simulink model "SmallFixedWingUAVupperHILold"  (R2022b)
settings: Solver=FixedStepDiscrete  StartTime=0.0  StopTime=inf  FixedStep=1/150  RelTol=1e-3
model workspace: external: MAT-File (data not in the file)
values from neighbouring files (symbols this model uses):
  env = struct    [InitDatactrl.m]
  uav = struct    [InitDatactrl.m]    (also in InitDatactrldf.m)
  x = x + points(1, i) * k(i) * ft    [bezir_n.m]
undefined symbols (not defined in the file or in its folder): current_a, current_filtered_a, DiscIntNeverNeededParam, remaining, RGBLED_COLOR_ENUM, RGBLED_MODE_ENUM, voltage_filtered_v, voltage_v
libraries: simulink x10, pixhawk_slib_sensors_actuators x6, pixhawk_slib_uORB_RW x5

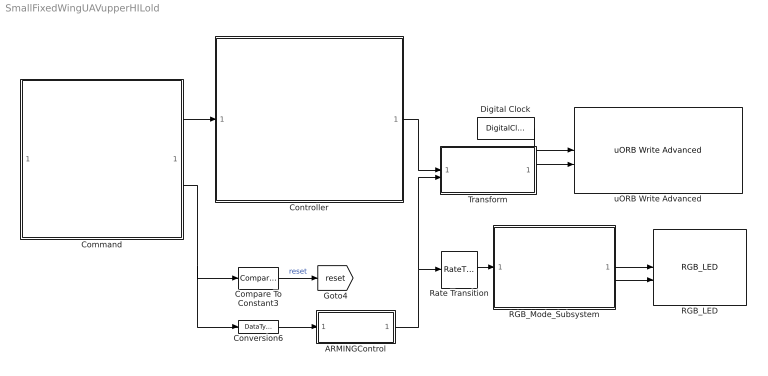
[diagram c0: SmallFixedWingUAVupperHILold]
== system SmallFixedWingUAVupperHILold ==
  ARMINGControl : Subsystem
  Command : Subsystem
  Compare To Constant3 : simulink/Logic and Bit Operations/Compare To Constant  relop=<=  const=1100  OutDataTypeStr=boolean
  Controller : Subsystem
  Conversion6 : DataTypeConversion  OutDataTypeStr=double
  Digital Clock : DigitalClock  SampleTime=-1
  RGB_LED : pixhawk_slib_sensors_actuators/RGB_LED
  RGB_Mode_Subsystem : Subsystem
  Rate Transition : RateTransition  OutPortSampleTime=1
  Transform : Subsystem
  uORB Write Advanced : pixhawk_slib_uORB_RW/uORB Write Advanced  Ts=0  uORB_AdvtQueue=on  uORB_FieldEnabledArr="0  0  0  1  0  0  0  0  0  0  0"  uORB_Topic_str=0  uORB_Struct_DT="[1  1  1  1  1]"  BlockInputCount=5  uORB_StructParams="[\"voltage_v\",\"voltage_filtered_v\",\"current_a\",\"current_filtered_a\",\"remaining\"]"  uORB_PortSizes="[1  1  1  1]"  MsgSizeOf=0  MW_update=true
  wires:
  Digital Clock/1 -> uORB Write Advanced/1
  RGB_Mode_Subsystem/1(RGB_MODE) -> RGB_LED/1
  Rate Transition/1 -> RGB_Mode_Subsystem/1(ARM_STATE)
  ARMINGControl/1(Out1) -> Transform/2(Arm), Rate Transition/1
  RGB_Mode_Subsystem/2(RGB_COLOR) -> RGB_LED/2
  Conversion6/1 -> ARMINGControl/1(In1)
  Compare To Constant3/1 -> [reset]  "reset"
  Transform/1(PWMOuput) -> uORB Write Advanced/2
  Controller/1(Actuator) -> Transform/1(ActuatorCmd)
  Command/2(Arm) -> Conversion6/1, Compare To Constant3/1
  Command/1(Command) -> Controller/1(Command)

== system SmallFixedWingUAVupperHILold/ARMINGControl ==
  In1 : Inport
  Compare To Constant3 : simulink/Logic and Bit Operations/Compare To Constant  relop=>=  const=uint16(1500)  OutDataTypeStr=boolean
  Out1 : Outport  VectorParamsAs1DForOutWhenUnconnected=off
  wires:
  Compare To Constant3/1 -> Out1/1
  In1/1 -> Compare To Constant3/1

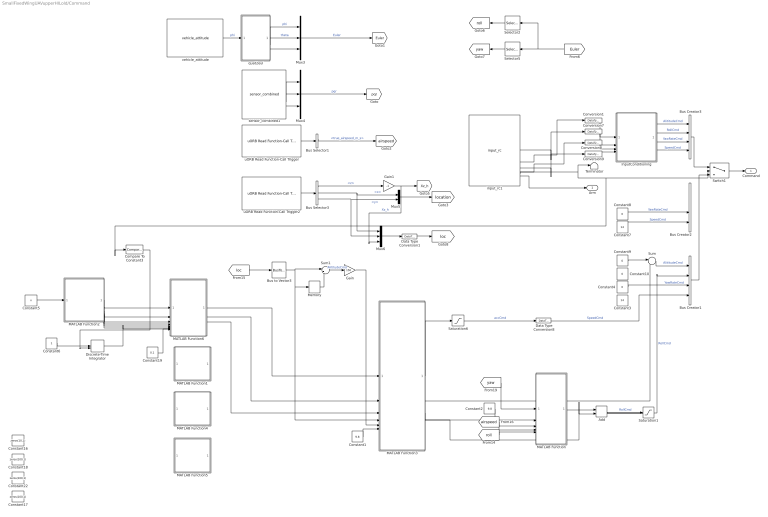
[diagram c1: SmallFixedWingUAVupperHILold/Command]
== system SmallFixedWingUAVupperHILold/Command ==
  Add : Sum
  Bus Creator1 : BusCreator  Inputs=4
  Bus Creator2 : BusCreator  Inputs=4
  Bus Creator3 : BusCreator  Inputs=4
  Bus Selector1 : BusSelector  OutputSignals=true_airspeed_m_s
  Bus Selector3 : BusSelector  OutputSignals=z,x,y
  Bus to Vector3 : BusToVector
  Compare To Constant3 : simulink/Logic and Bit Operations/Compare To Constant  relop=>=  const=uint16(1500)  OutDataTypeStr=boolean
  Constant1 : Constant  Value=9.8
  Constant{4,8..10} (4 alike) : Constant  Value=0  SampleTime=-1
  Constant16 : Constant  Value=zeros(10,1)
  Constant17 : Constant  Value=zeros(100,1)
  Constant18 : Constant  Value=zeros(100,1)
  Constant19 : Constant  Value=0.1
  Constant2 : Constant  Value=9.8  SampleTime=-1
  Constant22 : Constant  Value=zeros(100,1)
  Constant3 : Constant  Value=14  SampleTime=-1
  Constant5 : Constant  Value=x
  Constant6 : Constant
  Constant7 : Constant  Value=14  SampleTime=-1
  Conversion{1,7..9} (4 alike) : DataTypeConversion  OutDataTypeStr=double
  Data Type Conversion1 : DataTypeConversion  OutDataTypeStr=double
  Data Type Conversion8 : DataTypeConversion  OutDataTypeStr=single
  Discrete-Time Integrator : DiscreteIntegrator  ExternalReset=either  SampleTime=-1  ICPrevOutput=DiscIntNeverNeededParam  ICPrevScaledInput=DiscIntNeverNeededParam
  Gain : Gain  Gain=150
  Gain1 : Gain  Gain=-1
  InputConditioning : Subsystem
  MATLAB Function : MATLAB Function  TreatAsAtomicUnit=on
  MATLAB Function1 : MATLAB Function  Commented=on  TreatAsAtomicUnit=on
  MATLAB Function2 : MATLAB Function  TreatAsAtomicUnit=on
  MATLAB Function3 : MATLAB Function  TreatAsAtomicUnit=on
  MATLAB Function4 : MATLAB Function  Commented=on  TreatAsAtomicUnit=on
  MATLAB Function5 : MATLAB Function  Commented=on  TreatAsAtomicUnit=on
  MATLAB Function6 : MATLAB Function  TreatAsAtomicUnit=on
  Memory : Memory  InheritSampleTime=on
  Mux3 : Mux  Inputs=3
  Mux4 : Mux  Inputs=3
  Mux5 : Mux  Inputs=2
  Mux6 : Mux  Inputs=3
  Saturation1 : Saturate  UpperLimit=0.4  LowerLimit=-0.4
  Saturation6 : Saturate  UpperLimit=10  LowerLimit=-10
  Selector2 : Selector  InputPortWidth=3  IndexOptions=Index vector (dialog)  Indices=1  OutputSizes=1
  Selector5 : Selector  InputPortWidth=3  IndexOptions=Index vector (dialog)  Indices=3  OutputSizes=1
  Sum : Sum  Inputs=|++
  Sum1 : Sum  Inputs=|+-
  Switch1 : Switch  Criteria=u2 > Threshold  Threshold=1500
  Terminator : Terminator
  input_rc1 : pixhawk_slib_sensors_actuators/input_rc  Description=|  sampletime=1/150  channel1=on  channel2=on  channel3=on  channel4=on  channel5=on  channel6=on  channel7=off  channel8=off  channel9=off  channel10=off  channel11=off  channel12=off  channel13=off  channel14=off  channel15=off  channel16=off  channel17=off  channel18=off  ch_count=off  rssi=off  rc_failsafe=off  rc_lost=off  rc_inputsource=off
      | RC Input Block
      | 
      | This block provides user input control to the model.
      | It uses the input_rc uORB topic.
      | 
      | The user has the ability to choose which channels are available as outputs from this block and also some optional outputs. These include 
      | Channels 1 through 18
      | double data type indicating the PWM value from the controller 
      | measured pulse widths for each of the supported channels 
      | Channel Count 
      | u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
  quat2eul : MATLAB Function  TreatAsAtomicUnit=on
  sensor_combined1 : pixhawk_slib_sensors_actuators/sensor_combined  Description=|  sampletime=1/150  show_mag=off  show_acc=off  show_gyro=on  show_baro=off  show_ts=off
      | Sensor Combined Block
      | 
      | This block enables access to the various sensors available on the px4fmu-v2 hardware.  
      | The user can use these signals in the Simulink control model.  
      | The sample time needs to be provided in the mask dialog.  
      | Optional output ports can also be selected.  
      | Refer to the sample model: px4demo_attitude_control.slx
      | 
      | Signal definitions: 
      | Magnetometer (x,y,z) - single values – Mag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
  uORB Read Function-Call Trigger : pixhawk_slib_uORB_RW/uORB Read Function-Call Trigger  uORB_Topic_str='airspeed'  BusObjVar=Bus: airspeed_SL  uORB_Interval=1  AsyncOutput=off  Fcn_call_select=Generate Function Call Signal  TaskName='Task1'  Poll_timeout=100  Ts=-1
  uORB Read Function-Call Trigger2 : pixhawk_slib_uORB_RW/uORB Read Function-Call Trigger  uORB_Topic_str='vehicle_local_position'  BusObjVar=Bus: vehicle_local_position_SL  uORB_Interval=1  AsyncOutput=off  Fcn_call_select=Generate Function Call Signal  TaskName='Task1'  Poll_timeout=100  Ts=-1
  vehicle_attitude : pixhawk_slib_sensors_actuators/vehicle_attitude  sampletime=1/150  show_r=off  show_p=off  show_y=off  show_q=on  show_ts=off
  Command : Outport  VectorParamsAs1DForOutWhenUnconnected=off
  Arm : Outport  Port=2  VectorParamsAs1DForOutWhenUnconnected=off
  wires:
  InputConditioning/3(yawRate_d) -> Bus Creator3/3  "YawRateCmd"
  Conversion9/1 -> InputConditioning/4(ch4)
  InputConditioning/2(Roll_d) -> Bus Creator3/2  "RollCmd"
  Constant8/1 -> Bus Creator2/3  "YawRateCmd"
  InputConditioning/4(Speed_d) -> Bus Creator3/4  "SpeedCmd"
  Conversion1/1 -> InputConditioning/1("ch1 ")
  InputConditioning/1(Altitude_d) -> Bus Creator3/1  "AlititudeCmd"
  input_rc1/5 -> Switch1/2, Compare To Constant3/1, Terminator/1
  Conversion8/1 -> InputConditioning/3(ch3)
  Constant7/1 -> Bus Creator2/4  "SpeedCmd"
  Bus Creator3/1 -> Switch1/1
  Conversion7/1 -> InputConditioning/2(ch2)
  Switch1/1 -> Command/1
  input_rc1/6 -> Arm/1
  MATLAB Function3/4(roll) -> Add/2
  Saturation6/1 -> Data Type Conversion8/1  "accCmd"
  [airspeed] -> MATLAB Function/4(V)
  MATLAB Function3/3(yaw) -> MATLAB Function/2(yawdes)
  Bus to Vector3/1 -> Sum1/1, Memory/1, MATLAB Function3/4(x)
  Constant2/1 -> MATLAB Function/3(g)
  Constant1/1 -> MATLAB Function3/6(g)
  MATLAB Function/1(roll) -> Add/1
  MATLAB Function3/1(av1) -> Saturation6/1
  [loc] -> Bus to Vector3/1
  [roll] -> MATLAB Function/5(rolldes)
  [yaw] -> MATLAB Function/1(yaw)
  sensor_combined1/3 -> Mux4/3
  Mux4/1 -> [pqr]  "pqr"
  Mux3/1 -> [Euler]  "Euler"
  quat2eul/1(phi) -> Mux3/1  "phi"
  uORB Read Function-Call Trigger/1 -> Bus Selector1/1
  Bus Selector1/1 -> [airspeed]  "<true_airspeed_m_s>"
  vehicle_attitude/1 -> quat2eul/1(q)  "phi"
  quat2eul/2(theta) -> Mux3/2  "theta"
  sensor_combined1/2 -> Mux4/2
  sensor_combined1/1 -> Mux4/1
  quat2eul/3(psi) -> Mux3/3
  Mux6/1 -> Data Type Conversion1/1
  Bus Selector3/2 -> Mux6/1, Mux5/1  "<x>"
  Bus Selector3/3 -> Mux6/2, Mux5/2  "<y>"
  Bus Selector3/1 -> Gain1/1  "<z>"
  Gain1/1 -> Mux6/3, [Xz_h]  "Xz_h"
  Mux5/1 -> [location]
  uORB Read Function-Call Trigger2/1 -> Bus Selector3/1
  Data Type Conversion1/1 -> [loc]
  Selector2/1 -> [roll]
  Selector5/1 -> [yaw]
  [Euler] -> Selector2/1, Selector5/1
  Add/1 -> Saturation1/1  "RollCmd"
  Sum/1 -> Bus Creator1/1  "AlititudeCmd"
  Constant4/1 -> Bus Creator1/3  "YawRateCmd"
  Constant9/1 -> Sum/1
  Data Type Conversion8/1 -> Bus Creator1/4  "SpeedCmd"
  Memory/1 -> Sum1/2
  Sum1/1 -> Gain/1  "AlititudeCmd"
  Gain/1 -> MATLAB Function3/5(dx)
  Constant5/1 -> MATLAB Function2/1(x)
  MATLAB Function3/2(Hz) -> Sum/2
  Constant19/1 -> MATLAB Function6/8(sample_tt)
  MATLAB Function2/1(xx) -> MATLAB Function6/1(x)
  MATLAB Function6/1(xdx) -> MATLAB Function3/1(xd)
  MATLAB Function6/2(vdv) -> MATLAB Function3/2(dxd)
  MATLAB Function6/3(ada) -> MATLAB Function3/3(ddxd)
  Constant6/1 -> Discrete-Time Integrator/1
  Discrete-Time Integrator/1 -> MATLAB Function6/7(t)
  MATLAB Function2/2(y) -> MATLAB Function6/2(y)
  MATLAB Function2/3(dx) -> MATLAB Function6/3(dx)
  MATLAB Function2/4(dy) -> MATLAB Function6/4(dy)
  MATLAB Function2/5(ddx) -> MATLAB Function6/5(ddx)
  MATLAB Function2/6(ddy) -> MATLAB Function6/6(ddy)
  Saturation1/1 -> Bus Creator1/2  "RollCmd"
  Compare To Constant3/1 -> Discrete-Time Integrator/2
  Bus Creator1/1 -> Switch1/3
  input_rc1/3 -> Conversion9/1
  input_rc1/4 -> Conversion8/1
  input_rc1/1 -> Conversion7/1
  input_rc1/2 -> Conversion1/1

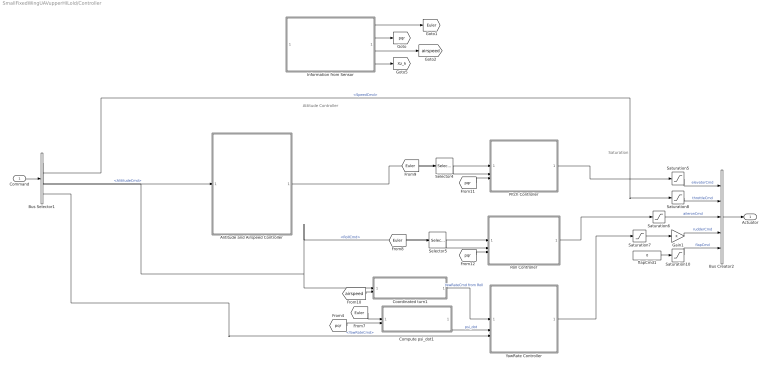
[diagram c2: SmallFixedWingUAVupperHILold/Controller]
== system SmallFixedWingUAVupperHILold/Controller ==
  note: Saturation
  note: Attitude Controller
  Command : Inport
  Alititude and Airspeed Controller : Subsystem
  Bus Creator2 : BusCreator  Inputs=5
  Bus Selector1 : BusSelector  OutputSignals=AlititudeCmd,SpeedCmd,RollCmd,YawRateCmd
  Compute psi_dot1 : Subsystem
  Coordinated turn1 : Subsystem
  Gain1 : Gain
  Information from Sensor : Subsystem
  Pitch Controller : Subsystem
  Roll Controller : Subsystem
  Saturation10 : Saturate  UpperLimit=uav.flap.max  LowerLimit=uav.flap.min
  Saturation5 : Saturate  UpperLimit=uav.elevator.max  LowerLimit=uav.elevator.min
  Saturation6 : Saturate  UpperLimit=uav.aileron.max  LowerLimit=uav.aileron.min
  Saturation7 : Saturate  UpperLimit=uav.rudder.max  LowerLimit=uav.rudder.min
  Saturation8 : Saturate  UpperLimit=uav.throttlepercent.max  LowerLimit=uav.throttlepercent.min
  Selector4 : Selector  InputPortWidth=3  IndexOptions=Index vector (dialog)  Indices=2  OutputSizes=1
  Selector5 : Selector  InputPortWidth=3  IndexOptions=Index vector (dialog)  Indices=1  OutputSizes=1
  YawRate Controller : Subsystem
  flapCmd1 : Constant  Value=0  OutDataTypeStr=double
  Actuator : Outport
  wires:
  Information from Sensor/1(Euler) -> [Euler]
  Information from Sensor/3(<true_airspeed_m_s>) -> [airspeed]
  Information from Sensor/2(pqr) -> [pqr]
  Information from Sensor/4(Xz_h) -> [Xz_h]
  Gain1/1 -> Bus Creator2/4  "rudderCmd"
  [pqr] -> Pitch Controller/3(pqr)
  [airspeed] -> Coordinated turn1/2(<airpseed>)
  Roll Controller/1(aileronCmd) -> Saturation6/1
  Bus Selector1/1 -> Alititude and Airspeed Controller/1(<AlititudeCmd>)  "<AlititudeCmd>"
  Saturation7/1 -> Gain1/1
  Bus Selector1/3 -> Coordinated turn1/1(<RollCmd>), Roll Controller/1(Roll cmd)  "<RollCmd>"
  Coordinated turn1/1(YawRateCmd) -> YawRate Controller/1(psi_dot Cmd)  "YawRateCmd from Roll"
  [Euler] -> Selector4/1
  Alititude and Airspeed Controller/1(pitchout) -> Pitch Controller/1(Pitch cmd)
  Pitch Controller/1(elevatorCmd) -> Saturation5/1
  Saturation8/1 -> Bus Creator2/2  "throttleCmd"
  Command/1 -> Bus Selector1/1
  flapCmd1/1 -> Saturation10/1
  Compute psi_dot1/1(psi_dot) -> YawRate Controller/2(psi_dot)  "psi_dot"
  [Euler] -> Selector5/1
  Bus Selector1/4 -> YawRate Controller/3(<YawRateCmd>)  "<YawRateCmd>"
  Saturation6/1 -> Bus Creator2/3  "aileronCmd"
  [pqr] -> Compute psi_dot1/2(G)
  Selector4/1 -> Pitch Controller/2(Pitch act)
  YawRate Controller/1(rudderCmd) -> Saturation7/1
  [pqr] -> Roll Controller/3(pqr)
  Selector5/1 -> Roll Controller/2(Roll act)
  Saturation5/1 -> Bus Creator2/1  "elevatorCmd"
  [Euler] -> Compute psi_dot1/1(Euler)
  Saturation10/1 -> Bus Creator2/5  "flapCmd"
  Bus Creator2/1 -> Actuator/1
  Bus Selector1/2 -> Saturation8/1  "<SpeedCmd>"

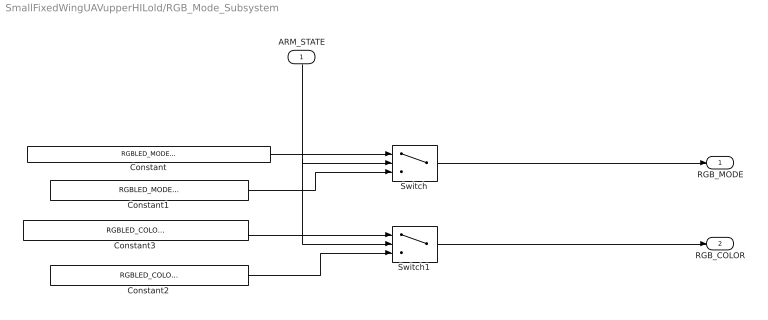
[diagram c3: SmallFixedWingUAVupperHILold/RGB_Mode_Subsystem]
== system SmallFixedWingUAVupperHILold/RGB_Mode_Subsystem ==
  ARM_STATE : Inport
  Constant : Constant  Value=RGBLED_MODE_ENUM.SL_MODE_BLINK_FAST  OutDataTypeStr=Enum: RGBLED_MODE_ENUM
  Constant1 : Constant  Value=RGBLED_MODE_ENUM.SL_MODE_BREATHE  OutDataTypeStr=Enum: RGBLED_MODE_ENUM
  Constant2 : Constant  Value=RGBLED_COLOR_ENUM.SL_COLOR_GREEN  OutDataTypeStr=Enum: RGBLED_COLOR_ENUM
  Constant3 : Constant  Value=RGBLED_COLOR_ENUM.SL_COLOR_BLUE  OutDataTypeStr=Enum: RGBLED_COLOR_ENUM
  Switch : Switch  Criteria=u2 ~= 0  Threshold=1500
  Switch1 : Switch  Criteria=u2 ~= 0  Threshold=1500
  RGB_MODE : Outport  VectorParamsAs1DForOutWhenUnconnected=off
  RGB_COLOR : Outport  Port=2  VectorParamsAs1DForOutWhenUnconnected=off
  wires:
  ARM_STATE/1 -> Switch1/2, Switch/2
  Constant/1 -> Switch/1
  Constant1/1 -> Switch/3
  Switch/1 -> RGB_MODE/1
  Constant3/1 -> Switch1/1
  Constant2/1 -> Switch1/3
  Switch1/1 -> RGB_COLOR/1

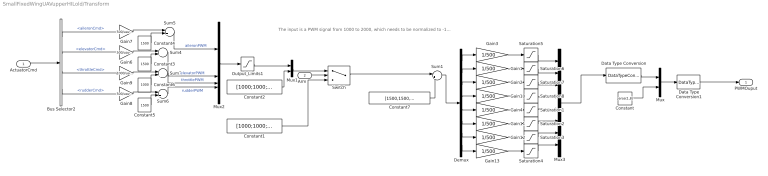
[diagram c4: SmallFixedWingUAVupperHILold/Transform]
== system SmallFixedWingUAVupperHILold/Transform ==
  note: The input is a PWM signal from 1000 to 2000, which needs to be normalized to -1~1.
  ActuatorCmd : Inport
  Arm : Inport  Port=2
  Bus Selector2 : BusSelector  OutputSignals=aileronCmd,elevatorCmd,throttleCmd,rudderCmd
  Constant : Constant  Value=zeros(1,8)
  Constant1 : Constant  Value=[1000;1000;1000;1000;1000;1000;1000;1000]
  Constant2 : Constant  Value=[1000;1000;1000;1000]
  Constant3 : Constant  Value=1500
  Constant4 : Constant  Value=1500
  Constant5 : Constant  Value=1500
  Constant6 : Constant  Value=1000
  Constant7 : Constant  Value=[1500,1500,1500,1500,1500,1500,1500,1500]
  Data Type Conversion : DataTypeConversion  OutDataTypeStr=double
  Data Type Conversion1 : DataTypeConversion  OutDataTypeStr=single
  Demux : Demux  Outputs=8
  Gain{1..4,10..13} (8 alike) : Gain  Gain=1/500
  Gain6 : Gain  Gain=500/uav.controlsurfacemax
  Gain7 : Gain  Gain=500/uav.controlsurfacemax
  Gain8 : Gain  Gain=500/uav.controlsurfacemax
  Gain9 : Gain  Gain=1000/uav.throttlepercent.max
  Mux : Mux  Inputs=2
  Mux1 : Mux  Inputs=2
  Mux2 : Mux
  Mux3 : Mux  Inputs=8
  Output_Limits1 : Saturate  UpperLimit=2000  LowerLimit=1000
  Saturation{1..8} (8 alike) : Saturate  UpperLimit=1  LowerLimit=-1
  Sum1 : Sum  Inputs=|+-
  Sum{4..7} (4 alike) : Sum  Inputs=|++
  Switch : Switch  Criteria=u2 > Threshold  Threshold=0.5
  PWMOuput : Outport  VectorParamsAs1DForOutWhenUnconnected=off
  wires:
  Constant2/1 -> Mux1/2
  Sum6/1 -> Mux2/4  "rudderPWM"
  Data Type Conversion/1 -> Mux/1
  Bus Selector2/4 -> Gain8/1  "<rudderCmd>"
  Bus Selector2/2 -> Gain6/1  "<elevatorCmd>"
  Constant3/1 -> Sum4/2
  Gain6/1 -> Sum4/1
  Bus Selector2/3 -> Gain9/1  "<throttleCmd>"
  Bus Selector2/1 -> Gain7/1  "<aileronCmd>"
  Constant/1 -> Mux/2
  Gain8/1 -> Sum6/1
  Sum7/1 -> Mux2/3  "throttlePWM"
  Constant1/1 -> Switch/3
  Mux1/1 -> Switch/1
  Output_Limits1/1 -> Mux1/1
  Constant5/1 -> Sum6/2
  Sum5/1 -> Mux2/1  "aileronPWM"
  Sum4/1 -> Mux2/2  "elevatorPWM"
  Constant6/1 -> Sum7/2
  Mux2/1 -> Output_Limits1/1
  Gain7/1 -> Sum5/1
  Mux/1 -> Data Type Conversion1/1
  Gain9/1 -> Sum7/1
  Constant4/1 -> Sum5/2
  Arm/1 -> Switch/2
  ActuatorCmd/1 -> Bus Selector2/1
  Data Type Conversion1/1 -> PWMOuput/1
  Demux/1 -> Gain3/1
  Saturation6/1 -> Mux3/2
  Saturation5/1 -> Mux3/1
  Gain1/1 -> Saturation6/1
  Sum1/1 -> Demux/1
  Saturation8/1 -> Mux3/4
  Gain2/1 -> Saturation7/1
  Demux/4 -> Gain10/1
  Gain3/1 -> Saturation5/1
  Demux/2 -> Gain1/1
  Saturation7/1 -> Mux3/3
  Demux/3 -> Gain2/1
  Gain10/1 -> Saturation8/1
  Constant7/1 -> Sum1/2
  Demux/7 -> Gain12/1
  Demux/6 -> Gain11/1
  Demux/5 -> Gain4/1
  Demux/8 -> Gain13/1
  Gain4/1 -> Saturation1/1
  Saturation1/1 -> Mux3/5
  Gain11/1 -> Saturation2/1
  Saturation2/1 -> Mux3/6
  Gain12/1 -> Saturation3/1
  Saturation3/1 -> Mux3/7
  Gain13/1 -> Saturation4/1
  Saturation4/1 -> Mux3/8
  Switch/1 -> Sum1/1
  Mux3/1 -> Data Type Conversion/1

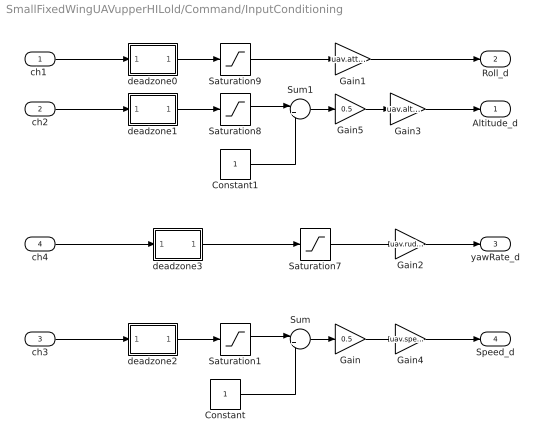
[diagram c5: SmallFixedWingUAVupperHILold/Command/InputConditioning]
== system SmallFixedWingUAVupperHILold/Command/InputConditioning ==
  "ch1 " : Inport
  ch2 : Inport  Port=2
  ch3 : Inport  Port=3
  ch4 : Inport  Port=4
  Constant : Constant
  Constant1 : Constant
  Gain : Gain  Gain=0.5
  Gain1 : Gain  Gain=uav.attitudectrlmax.roll  OutDataTypeStr=Inherit: Inherit via back propagation
  Gain2 : Gain  Gain=uav.rudder.max
  Gain3 : Gain  Gain=uav.altitude.max  OutDataTypeStr=Inherit: Inherit via back propagation
  Gain4 : Gain  Gain=uav.speed.max
  Gain5 : Gain  Gain=0.5
  Saturation{1,7..9} (4 alike) : Saturate  UpperLimit=1  LowerLimit=-1
  Sum : Sum  Inputs=|++
  Sum1 : Sum  Inputs=|++
  deadzone0 : MATLAB Function  TreatAsAtomicUnit=on
  deadzone1 : MATLAB Function  TreatAsAtomicUnit=on
  deadzone2 : MATLAB Function  TreatAsAtomicUnit=on
  deadzone3 : MATLAB Function  TreatAsAtomicUnit=on
  Altitude_d : Outport  VectorParamsAs1DForOutWhenUnconnected=off
  Roll_d : Outport  Port=2  VectorParamsAs1DForOutWhenUnconnected=off
  yawRate_d : Outport  Port=3  VectorParamsAs1DForOutWhenUnconnected=off
  Speed_d : Outport  Port=4  VectorParamsAs1DForOutWhenUnconnected=off
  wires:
  deadzone2/1(y) -> Saturation1/1
  ch3/1 -> deadzone2/1(u)
  deadzone1/1(y) -> Saturation8/1
  Gain/1 -> Gain4/1
  deadzone0/1(y) -> Saturation9/1
  "ch1 "/1 -> deadzone0/1(u)
  ch2/1 -> deadzone1/1(u)
  Saturation9/1 -> Gain1/1
  Saturation8/1 -> Sum1/1
  Constant/1 -> Sum/2
  Sum/1 -> Gain/1
  Gain1/1 -> Roll_d/1
  Gain3/1 -> Altitude_d/1
  Saturation7/1 -> Gain2/1
  deadzone3/1(y) -> Saturation7/1
  ch4/1 -> deadzone3/1(u)
  Gain2/1 -> yawRate_d/1
  Saturation1/1 -> Sum/1
  Gain4/1 -> Speed_d/1
  Gain5/1 -> Gain3/1
  Constant1/1 -> Sum1/2
  Sum1/1 -> Gain5/1

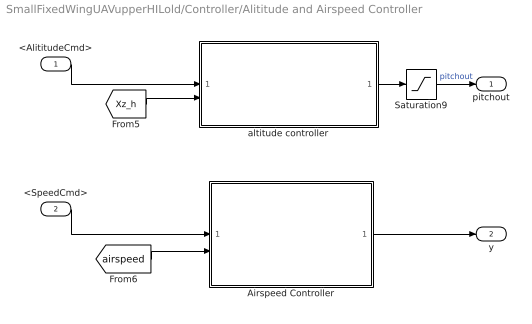
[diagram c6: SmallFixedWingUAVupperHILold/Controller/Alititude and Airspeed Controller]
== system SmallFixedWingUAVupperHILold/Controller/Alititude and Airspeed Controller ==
  <AlititudeCmd> : Inport
  <SpeedCmd> : Inport  Port=2
  Airspeed Controller : Subsystem
  Saturation9 : Saturate  UpperLimit=uav.attitudectrlmax.pitch  LowerLimit=-uav.attitudectrlmax.pitch
  altitude controller : Subsystem
  pitchout : Outport
  y : Outport  Port=2
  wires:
  <AlititudeCmd>/1 -> altitude controller/1(Alititude cmd)
  [airspeed] -> Airspeed Controller/2(speed act)
  altitude controller/1(pitchout) -> Saturation9/1
  Saturation9/1 -> pitchout/1  "pitchout"
  [Xz_h] -> altitude controller/2(Alititude act)
  Airspeed Controller/1(y) -> y/1
  <SpeedCmd>/1 -> Airspeed Controller/1(Speed cmd)

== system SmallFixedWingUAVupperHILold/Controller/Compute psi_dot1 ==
  Euler : Inport
  G : Inport  Port=2
  Mux1 : Mux  Inputs=2
  psidot : Fcn  Expr=(u[5]*sin(u[1])+u[6]*cos(u[1]))/cos(u[2])
  psi_dot : Outport  Unit=rad/S  VectorParamsAs1DForOutWhenUnconnected=off
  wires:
  G/1 -> Mux1/2
  psidot/1 -> psi_dot/1  "psi_dot"
  Mux1/1 -> psidot/1
  Euler/1 -> Mux1/1

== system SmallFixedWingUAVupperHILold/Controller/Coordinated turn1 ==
  <RollCmd> : Inport
  <airpseed> : Inport  Port=2
  Divide : Product  Inputs=*/*
  Trigonometric Function : Trigonometry  Operator=tan
  env.ISA_g : Constant  Value=env.ISA_g
  YawRateCmd : Outport  VectorParamsAs1DForOutWhenUnconnected=off
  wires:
  Trigonometric Function/1 -> Divide/1
  <RollCmd>/1 -> Trigonometric Function/1
  env.ISA_g/1 -> Divide/3
  Divide/1 -> YawRateCmd/1  "YawRateCmd from Roll"
  <airpseed>/1 -> Divide/2

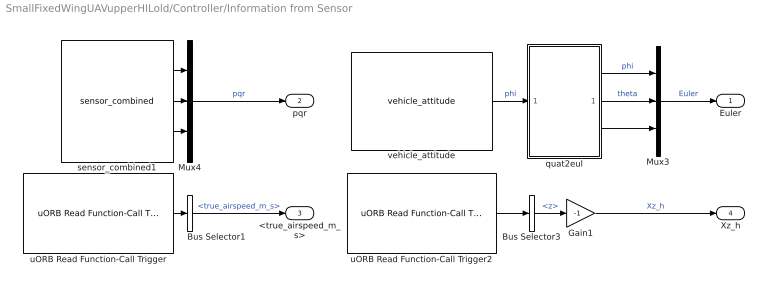
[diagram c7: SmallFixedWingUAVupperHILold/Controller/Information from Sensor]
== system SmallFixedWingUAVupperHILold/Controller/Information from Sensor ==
  Bus Selector1 : BusSelector  OutputSignals=true_airspeed_m_s
  Bus Selector3 : BusSelector  OutputSignals=z
  Gain1 : Gain  Gain=-1
  Mux3 : Mux  Inputs=3
  Mux4 : Mux  Inputs=3
  quat2eul : MATLAB Function  TreatAsAtomicUnit=on
  sensor_combined1 : pixhawk_slib_sensors_actuators/sensor_combined  Description=|  sampletime=1/150  show_mag=off  show_acc=off  show_gyro=on  show_baro=off  show_ts=off
      | Sensor Combined Block
      | 
      | This block enables access to the various sensors available on the px4fmu-v2 hardware.  
      | The user can use these signals in the Simulink control model.  
      | The sample time needs to be provided in the mask dialog.  
      | Optional output ports can also be selected.  
      | Refer to the sample model: px4demo_attitude_control.slx
      | 
      | Signal definitions: 
      | Magnetometer (x,y,z) - single values – Mag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
  uORB Read Function-Call Trigger : pixhawk_slib_uORB_RW/uORB Read Function-Call Trigger  uORB_Topic_str='airspeed'  BusObjVar=Bus: airspeed_SL  uORB_Interval=1  AsyncOutput=off  Fcn_call_select=Generate Function Call Signal  TaskName='Task1'  Poll_timeout=100  Ts=-1
  uORB Read Function-Call Trigger2 : pixhawk_slib_uORB_RW/uORB Read Function-Call Trigger  uORB_Topic_str='vehicle_local_position'  BusObjVar=Bus: vehicle_local_position_SL  uORB_Interval=1  AsyncOutput=off  Fcn_call_select=Generate Function Call Signal  TaskName='Task1'  Poll_timeout=100  Ts=-1
  vehicle_attitude : pixhawk_slib_sensors_actuators/vehicle_attitude  sampletime=1/150  show_r=off  show_p=off  show_y=off  show_q=on  show_ts=off
  Euler : Outport  VectorParamsAs1DForOutWhenUnconnected=off
  pqr : Outport  Port=2  VectorParamsAs1DForOutWhenUnconnected=off
  <true_airspeed_m_s> : Outport  Port=3  VectorParamsAs1DForOutWhenUnconnected=off
  Xz_h : Outport  Port=4  VectorParamsAs1DForOutWhenUnconnected=off
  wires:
  sensor_combined1/2 -> Mux4/2
  Mux4/1 -> pqr/1  "pqr"
  Mux3/1 -> Euler/1  "Euler"
  Gain1/1 -> Xz_h/1  "Xz_h"
  Bus Selector1/1 -> <true_airspeed_m_s>/1  "<true_airspeed_m_s>"
  quat2eul/3(psi) -> Mux3/3
  quat2eul/1(phi) -> Mux3/1  "phi"
  vehicle_attitude/1 -> quat2eul/1(q)  "phi"
  uORB Read Function-Call Trigger/1 -> Bus Selector1/1
  uORB Read Function-Call Trigger2/1 -> Bus Selector3/1
  sensor_combined1/3 -> Mux4/3
  sensor_combined1/1 -> Mux4/1
  Bus Selector3/1 -> Gain1/1  "<z>"
  quat2eul/2(theta) -> Mux3/2  "theta"

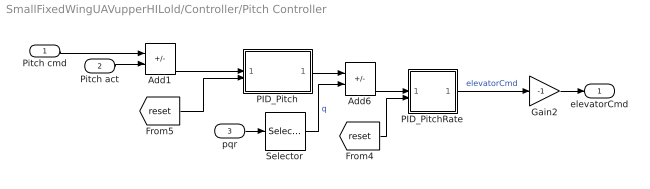
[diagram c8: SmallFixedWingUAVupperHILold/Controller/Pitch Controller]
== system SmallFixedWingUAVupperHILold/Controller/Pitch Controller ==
  Pitch cmd : Inport
  Pitch act : Inport  Port=2
  pqr : Inport  Port=3
  Add1 : Sum  Inputs=+-
  Add6 : Sum  Inputs=+-
  Gain2 : Gain  Gain=-1
  PID_Pitch : Subsystem
  PID_PitchRate : Subsystem
  Selector : Selector  InputPortWidth=3  IndexOptions=Index vector (dialog)  Indices=2  OutputSizes=1
  elevatorCmd : Outport  VectorParamsAs1DForOutWhenUnconnected=off
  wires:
  PID_PitchRate/1(y) -> Gain2/1  "elevatorCmd"
  [reset] -> PID_PitchRate/2(reset_i)
  [reset] -> PID_Pitch/2(reset_i)
  Add1/1 -> PID_Pitch/1(e_theta)
  Add6/1 -> PID_PitchRate/1(x)
  Pitch act/1 -> Add1/2
  Gain2/1 -> elevatorCmd/1
  Selector/1 -> Add6/2  "q"
  PID_Pitch/1(qCmd) -> Add6/1
  pqr/1 -> Selector/1
  Pitch cmd/1 -> Add1/1

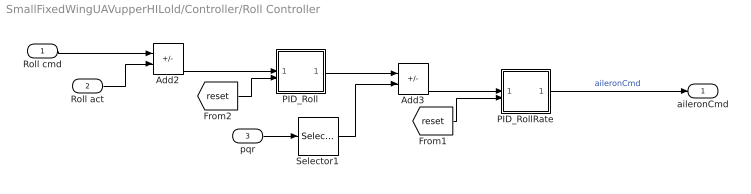
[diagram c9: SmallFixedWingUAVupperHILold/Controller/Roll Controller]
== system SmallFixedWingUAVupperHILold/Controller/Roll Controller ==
  Roll cmd : Inport
  Roll act : Inport  Port=2
  pqr : Inport  Port=3
  Add2 : Sum  Inputs=+-
  Add3 : Sum  Inputs=+-
  PID_Roll : Subsystem
  PID_RollRate : Subsystem
  Selector1 : Selector  InputPortWidth=3  IndexOptions=Index vector (dialog)  Indices=1  OutputSizes=1
  aileronCmd : Outport  VectorParamsAs1DForOutWhenUnconnected=off
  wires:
  PID_RollRate/1(y) -> aileronCmd/1  "aileronCmd"
  Add2/1 -> PID_Roll/1(x)
  Add3/1 -> PID_RollRate/1(x)
  Selector1/1 -> Add3/2
  [reset] -> PID_RollRate/2(reset_i)
  [reset] -> PID_Roll/2(reset_i)
  pqr/1 -> Selector1/1
  Roll act/1 -> Add2/2
  PID_Roll/1(y) -> Add3/1
  Roll cmd/1 -> Add2/1

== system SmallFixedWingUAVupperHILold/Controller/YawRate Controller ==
  psi_dot Cmd : Inport
  psi_dot : Inport  Port=2
  <YawRateCmd> : Inport  Port=3
  Add4 : Sum  Inputs=+-
  PID_YawRate : Subsystem
  Sum2 : Sum  Inputs=++|
  rudderCmd : Outport  VectorParamsAs1DForOutWhenUnconnected=off
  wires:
  Sum2/1 -> rudderCmd/1  "rudderCmd"
  Add4/1 -> PID_YawRate/1(x)
  [reset] -> PID_YawRate/2(reset_i)
  PID_YawRate/1(y) -> Sum2/2
  psi_dot/1 -> Add4/2
  psi_dot Cmd/1 -> Add4/1

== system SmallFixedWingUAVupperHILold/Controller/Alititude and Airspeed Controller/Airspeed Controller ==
  Speed cmd : Inport
  speed act : Inport  Port=2
  Add7 : Sum  Inputs=+-
  PID_Speed : Subsystem
  y : Outport
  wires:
  [reset] -> PID_Speed/2(reset_i)
  PID_Speed/1(y) -> y/1
  Add7/1 -> PID_Speed/1(x)  "speederror"
  speed act/1 -> Add7/2
  Speed cmd/1 -> Add7/1

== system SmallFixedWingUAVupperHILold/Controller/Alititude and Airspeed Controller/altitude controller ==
  Alititude cmd : Inport
  Alititude act : Inport  Port=2
  Add8 : Sum  Inputs=+-
  PID_Altitude : Subsystem
  pitchout : Outport
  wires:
  [reset] -> PID_Altitude/2(reset_i)
  PID_Altitude/1(y) -> pitchout/1  "pitchout"
  Add8/1 -> PID_Altitude/1(x)
  Alititude act/1 -> Add8/2
  Alititude cmd/1 -> Add8/1

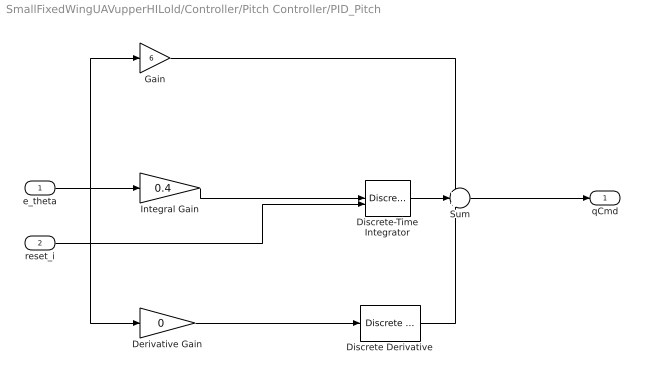
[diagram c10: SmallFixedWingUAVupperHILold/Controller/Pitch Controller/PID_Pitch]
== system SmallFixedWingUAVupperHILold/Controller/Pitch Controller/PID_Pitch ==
  e_theta : Inport
  reset_i : Inport  Port=2
  Derivative Gain : Gain  DisableCoverage=on  Gain=0  ParamMin=-100  ParamMax=100  OutMin=-100  OutMax=100
  Discrete Derivative : simulink/Discrete/Discrete Derivative  gainval=1.0  ICPrevScaledInput=0.0  OutMin=[]  OutMax=[]  OutDataType=fixdt(1, 16)  OutScaling=2^-10  DoSatur=off
  Discrete-Time Integrator : DiscreteIntegrator  ExternalReset=either  SampleTime=-1  ICPrevOutput=DiscIntNeverNeededParam  ICPrevScaledInput=DiscIntNeverNeededParam
  Gain : Gain  Gain=6
  Integral Gain : Gain  DisableCoverage=on  Gain=0.4
  Sum : Sum  Inputs=+++
  qCmd : Outport  InitialOutput=0  VectorParamsAs1DForOutWhenUnconnected=off
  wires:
  e_theta/1 -> Gain/1, Integral Gain/1, Derivative Gain/1
  Integral Gain/1 -> Discrete-Time Integrator/1
  Derivative Gain/1 -> Discrete Derivative/1
  Gain/1 -> Sum/1
  Sum/1 -> qCmd/1
  Discrete Derivative/1 -> Sum/3
  Discrete-Time Integrator/1 -> Sum/2
  reset_i/1 -> Discrete-Time Integrator/2

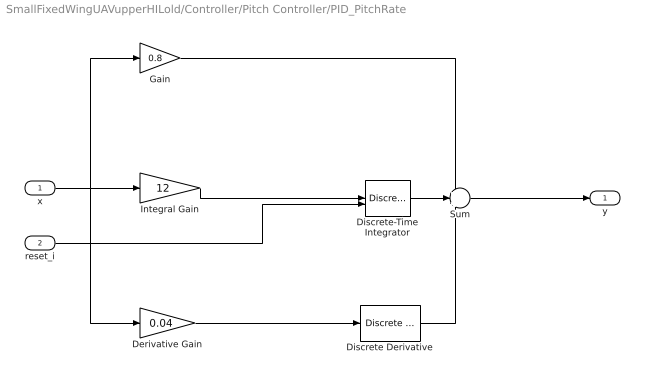
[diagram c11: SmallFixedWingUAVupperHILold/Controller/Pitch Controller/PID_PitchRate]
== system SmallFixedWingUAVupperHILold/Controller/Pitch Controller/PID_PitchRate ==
  x : Inport
  reset_i : Inport  Port=2
  Derivative Gain : Gain  DisableCoverage=on  Gain=0.04  ParamMin=-100  ParamMax=100  OutMin=-100  OutMax=100
  Discrete Derivative : simulink/Discrete/Discrete Derivative  gainval=1.0  ICPrevScaledInput=0.0  OutMin=[]  OutMax=[]  OutDataType=fixdt(1, 16)  OutScaling=2^-10  DoSatur=off
  Discrete-Time Integrator : DiscreteIntegrator  ExternalReset=either  SampleTime=-1  LimitOutput=on  UpperSaturationLimit=0.3  LowerSaturationLimit=-0.3  ICPrevOutput=DiscIntNeverNeededParam  ICPrevScaledInput=DiscIntNeverNeededParam
  Gain : Gain  Gain=0.8
  Integral Gain : Gain  DisableCoverage=on  Gain=12
  Sum : Sum  Inputs=+++
  y : Outport  InitialOutput=0  VectorParamsAs1DForOutWhenUnconnected=off
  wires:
  reset_i/1 -> Discrete-Time Integrator/2
  Discrete-Time Integrator/1 -> Sum/2
  Discrete Derivative/1 -> Sum/3
  Sum/1 -> y/1
  Gain/1 -> Sum/1
  Derivative Gain/1 -> Discrete Derivative/1
  Integral Gain/1 -> Discrete-Time Integrator/1
  x/1 -> Derivative Gain/1, Integral Gain/1, Gain/1

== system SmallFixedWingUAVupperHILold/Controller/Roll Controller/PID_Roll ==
  x : Inport
  reset_i : Inport  Port=2
  Derivative Gain : Gain  DisableCoverage=on  Gain=0  ParamMin=-100  ParamMax=100  OutMin=-100  OutMax=100
  Discrete Derivative : simulink/Discrete/Discrete Derivative  gainval=1.0  ICPrevScaledInput=0.0  OutMin=[]  OutMax=[]  OutDataType=fixdt(1, 16)  OutScaling=2^-10  DoSatur=off
  Discrete-Time Integrator : DiscreteIntegrator  ExternalReset=either  SampleTime=-1  ICPrevOutput=DiscIntNeverNeededParam  ICPrevScaledInput=DiscIntNeverNeededParam
  Gain : Gain  Gain=9
  Integral Gain : Gain  DisableCoverage=on  Gain=0.4
  Sum : Sum  Inputs=+++
  y : Outport  InitialOutput=0  VectorParamsAs1DForOutWhenUnconnected=off
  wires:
  reset_i/1 -> Discrete-Time Integrator/2
  Discrete-Time Integrator/1 -> Sum/2
  Discrete Derivative/1 -> Sum/3
  Sum/1 -> y/1
  Gain/1 -> Sum/1
  Derivative Gain/1 -> Discrete Derivative/1
  Integral Gain/1 -> Discrete-Time Integrator/1
  x/1 -> Derivative Gain/1, Integral Gain/1, Gain/1

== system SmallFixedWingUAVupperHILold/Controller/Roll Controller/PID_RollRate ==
  x : Inport
  reset_i : Inport  Port=2
  Derivative Gain : Gain  DisableCoverage=on  Gain=0.01  ParamMin=-100  ParamMax=100  OutMin=-100  OutMax=100
  Discrete Derivative : simulink/Discrete/Discrete Derivative  gainval=1.0  ICPrevScaledInput=0.0  OutMin=[]  OutMax=[]  OutDataType=fixdt(1, 16)  OutScaling=2^-10  DoSatur=off
  Discrete-Time Integrator : DiscreteIntegrator  ExternalReset=either  SampleTime=-1  LimitOutput=on  UpperSaturationLimit=0.3  LowerSaturationLimit=-0.3  ICPrevOutput=DiscIntNeverNeededParam  ICPrevScaledInput=DiscIntNeverNeededParam
  Gain : Gain  Gain=0.8
  Integral Gain : Gain  DisableCoverage=on  Gain=2
  Sum : Sum  Inputs=+++
  y : Outport  InitialOutput=0  VectorParamsAs1DForOutWhenUnconnected=off
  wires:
  x/1 -> Gain/1, Integral Gain/1, Derivative Gain/1
  Integral Gain/1 -> Discrete-Time Integrator/1
  Derivative Gain/1 -> Discrete Derivative/1
  Gain/1 -> Sum/1
  Sum/1 -> y/1
  Discrete Derivative/1 -> Sum/3
  Discrete-Time Integrator/1 -> Sum/2
  reset_i/1 -> Discrete-Time Integrator/2

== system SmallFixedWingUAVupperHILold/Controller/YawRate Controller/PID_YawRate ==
  x : Inport
  reset_i : Inport  Port=2
  Derivative Gain : Gain  DisableCoverage=on  Gain=0.3  ParamMin=-100  ParamMax=100  OutMin=-100  OutMax=100
  Discrete Derivative : simulink/Discrete/Discrete Derivative  gainval=1.0  ICPrevScaledInput=0.0  OutMin=[]  OutMax=[]  OutDataType=fixdt(1, 16)  OutScaling=2^-10  DoSatur=off
  Discrete-Time Integrator : DiscreteIntegrator  ExternalReset=either  SampleTime=-1  LimitOutput=on  UpperSaturationLimit=0.3  LowerSaturationLimit=-0.3  ICPrevOutput=DiscIntNeverNeededParam  ICPrevScaledInput=DiscIntNeverNeededParam
  Gain : Gain  Gain=4
  Integral Gain : Gain  DisableCoverage=on  Gain=3
  Sum : Sum  Inputs=+++
  y : Outport  InitialOutput=0  VectorParamsAs1DForOutWhenUnconnected=off
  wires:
  reset_i/1 -> Discrete-Time Integrator/2
  Discrete-Time Integrator/1 -> Sum/2
  Discrete Derivative/1 -> Sum/3
  Sum/1 -> y/1
  Gain/1 -> Sum/1
  Derivative Gain/1 -> Discrete Derivative/1
  Integral Gain/1 -> Discrete-Time Integrator/1
  x/1 -> Derivative Gain/1, Integral Gain/1, Gain/1

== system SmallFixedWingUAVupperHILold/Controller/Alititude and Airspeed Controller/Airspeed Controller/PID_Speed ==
  x : Inport
  reset_i : Inport  Port=2
  Derivative Gain : Gain  DisableCoverage=on  Gain=0.1  ParamMin=-100  ParamMax=100  OutMin=-100  OutMax=100
  Discrete Derivative : simulink/Discrete/Discrete Derivative  gainval=1.0  ICPrevScaledInput=0.0  OutMin=[]  OutMax=[]  OutDataType=fixdt(1, 16)  OutScaling=2^-10  DoSatur=off
  Discrete-Time Integrator : DiscreteIntegrator  ExternalReset=either  SampleTime=-1  UpperSaturationLimit=0.3  LowerSaturationLimit=-0.3  ICPrevOutput=DiscIntNeverNeededParam  ICPrevScaledInput=DiscIntNeverNeededParam
  Gain : Gain  Gain=0.5
  Integral Gain : Gain  DisableCoverage=on  Gain=0
  Sum : Sum  Inputs=+++
  y : Outport  InitialOutput=0  VectorParamsAs1DForOutWhenUnconnected=off
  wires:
  reset_i/1 -> Discrete-Time Integrator/2
  Discrete-Time Integrator/1 -> Sum/2
  Discrete Derivative/1 -> Sum/3
  Sum/1 -> y/1
  Gain/1 -> Sum/1
  Derivative Gain/1 -> Discrete Derivative/1
  Integral Gain/1 -> Discrete-Time Integrator/1
  x/1 -> Derivative Gain/1, Integral Gain/1, Gain/1

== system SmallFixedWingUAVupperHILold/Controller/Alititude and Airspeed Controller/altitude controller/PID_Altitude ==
  x : Inport
  reset_i : Inport  Port=2
  Derivative Gain : Gain  DisableCoverage=on  Gain=0  ParamMin=-100  ParamMax=100  OutMin=-100  OutMax=100
  Discrete Derivative : simulink/Discrete/Discrete Derivative  gainval=1.0  ICPrevScaledInput=0.0  OutMin=[]  OutMax=[]  OutDataType=fixdt(1, 16)  OutScaling=2^-10  DoSatur=off
  Discrete-Time Integrator : DiscreteIntegrator  ExternalReset=either  SampleTime=-1  ICPrevOutput=DiscIntNeverNeededParam  ICPrevScaledInput=DiscIntNeverNeededParam
  Gain : Gain  Gain=0.055
  Integral Gain : Gain  DisableCoverage=on  Gain=0
  Sum : Sum  Inputs=+++
  y : Outport  InitialOutput=0  VectorParamsAs1DForOutWhenUnconnected=off
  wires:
  x/1 -> Gain/1, Integral Gain/1, Derivative Gain/1
  Integral Gain/1 -> Discrete-Time Integrator/1
  Derivative Gain/1 -> Discrete Derivative/1
  Gain/1 -> Sum/1
  Sum/1 -> y/1
  Discrete Derivative/1 -> Sum/3
  Discrete-Time Integrator/1 -> Sum/2
  reset_i/1 -> Discrete-Time Integrator/2

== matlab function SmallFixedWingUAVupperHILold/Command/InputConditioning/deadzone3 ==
function y = fcn(u)
%Function description:
%  Control the range of the remote control input from RCMin to RCMax, and set
%  a dead zone with a dead zone size of ±deadZone,the output y is
%  normalized to 0~1.You can get the RC calibration parameters in QGC.
RCMin = 1100;
RCMax = 1900;
RCMid = (RCMin + RCMax)/2;
deadZoneRate = 0.05;
deadZone = deadZoneRate*(RCMax - RCMin);
k = 1/(RCMax - RCMid - deadZone);
%Limiting
if(u < RCMin)
    u = RCMin;
elseif(u > RCMax)
    u = RCMax;
end
%dead zone and normalize
 if(u > RCMid + deadZone)
    y = (u-RCMid - deadZone)*k;
 elseif(u < RCMid - deadZone)
     y = (u - RCMid + deadZone)*k;
 else
     y = 0;
 end

 end

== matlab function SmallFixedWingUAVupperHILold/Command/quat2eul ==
function [phi,theta,psi] = quat2eul(q)
% Conversion from Quaternion to Euler angles based on the PX4 Firmware
% v1.6.5 release.
% 
% Quaternion -> DCM -> Euler Angles
% INPUT:
%   q: Quaternion vector of the format: (a + bi + cj + dk)
% OUTPUT:
%   [phi,theta,psi]: Euler angles in radians.
% 
 
    a = q(1);
    b = q(2);
    c = q(3);
    d = q(4);

    aSq = a*a;
    bSq = b*b;
    cSq = c*c;
    dSq = d*d;

    d_pi2 = pi/2;

    % quaternion_to_dcm
    dcm00 = aSq + bSq - cSq - dSq;
    % dcm01 = 2*(b*c - a*d);
    dcm02 = 2*(a*c + b*d);
    dcm10 = 2*(b*c + a*d);
    % dcm11 = aSq - bSq + cSq - dSq;
    dcm12 = 2*(c*d - a*b);
    dcm20 = 2*(b*d - a*c);
    dcm21 = 2*(a*b + c*d);
    dcm22 = aSq - bSq - cSq + dSq;

    % dcm_to_euler
    theta = asin(-dcm20);
    if abs(theta - d_pi2) < 1.0e-3
        phi = single(0.0);
        psi = atan2(dcm12, dcm02);
    elseif abs(theta + d_pi2) < 1.0e-3
        phi = single(0.0);
        psi = atan2(-dcm12, -dcm02);
    else
        phi = atan2(dcm21, dcm22);
        psi = atan2(dcm10, dcm00);
    end

end

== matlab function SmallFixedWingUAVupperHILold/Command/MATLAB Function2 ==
function [xx,y,dx,dy,ddx,ddy]  = track(x)
%     index = int8(t/sample_tt);
%     if index <= 1
%         index = int8(1);
%     end
%     if index >= length(x)
%         index = int8(length(x));
%     end
    len = length(x)/6;

    xx = x(1:len);
    y = x(len+1:2*len);
    dx = x(2*len+1:3*len);
    dy = x(3*len+1:4*len);
    ddx = x(4*len+1:5*len);
    ddy = x(5*len+1:6*len);
end

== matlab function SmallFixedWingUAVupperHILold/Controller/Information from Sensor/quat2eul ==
function [phi,theta,psi] = quat2eul(q)
% Conversion from Quaternion to Euler angles based on the PX4 Firmware
% v1.6.5 release.
% 
% Quaternion -> DCM -> Euler Angles
% INPUT:
%   q: Quaternion vector of the format: (a + bi + cj + dk)
% OUTPUT:
%   [phi,theta,psi]: Euler angles in radians.
% 
 
    a = q(1);
    b = q(2);
    c = q(3);
    d = q(4);

    aSq = a*a;
    bSq = b*b;
    cSq = c*c;
    dSq = d*d;

    d_pi2 = pi/2;

    % quaternion_to_dcm
    dcm00 = aSq + bSq - cSq - dSq;
    % dcm01 = 2*(b*c - a*d);
    dcm02 = 2*(a*c + b*d);
    dcm10 = 2*(b*c + a*d);
    % dcm11 = aSq - bSq + cSq - dSq;
    dcm12 = 2*(c*d - a*b);
    dcm20 = 2*(b*d - a*c);
    dcm21 = 2*(a*b + c*d);
    dcm22 = aSq - bSq - cSq + dSq;

    % dcm_to_euler
    theta = asin(-dcm20);
    if abs(theta - d_pi2) < 1.0e-3
        phi = single(0.0);
        psi = atan2(dcm12, dcm02);
    elseif abs(theta + d_pi2) < 1.0e-3
        phi = single(0.0);
        psi = atan2(-dcm12, -dcm02);
    else
        phi = atan2(dcm21, dcm22);
        psi = atan2(dcm10, dcm00);
    end

end

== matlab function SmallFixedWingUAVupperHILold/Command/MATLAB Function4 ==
function vdv  = track(x,t,sample_tt)
%     index = int8(t/sample_tt);
%     if index <= 1
%         index = int8(1);
%     end
%     if index >= length(x)
%         index = int8(length(x));
%     end
    index = 1;
    dxx = x(index+300);
    dyy = x(index+400);

    vdv = [dxx;-dyy;0];
end

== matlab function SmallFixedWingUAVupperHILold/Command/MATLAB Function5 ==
function ada  = track(x,t,sample_tt)
%     index = int8(t/sample_tt);
%     if index <= 1
%         index = int8(1);
%     end
%     if index >= length(x)
%         index = int8(length(x));
%     end
    index = 10;
    ddxx = x(index+500);
    ddyy = x(index+600);

    ada = [ddxx;-ddyy;0];
end

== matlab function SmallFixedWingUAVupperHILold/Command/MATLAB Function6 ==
function [xdx,vdv,ada]  = track(x,y,dx,dy,ddx,ddy,t,sample_tt)
    index = int16(t/sample_tt);
    if index <= 1
        index = int16(1);
    end
    if index >= length(x)
        index = int16(length(x));
    end
    xx = x(index);
    yy = y(index);
    dxx = dx(index);
    dyy = dy(index);
    ddxx = ddx(index);
    ddyy = ddy(index);

    xdx = [xx;-yy;10];
    vdv = [dxx;-dyy;0];
    ada = [ddxx;-ddyy;0];
end

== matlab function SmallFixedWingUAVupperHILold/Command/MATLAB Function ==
function roll = fcn(yaw,yawdes,g,V,rolldes)
%     roll = yawrate*g*V;
    if yaw>pi
        yaw = yaw-2*pi;
    end
    yawrate = 2*(yawdes-yaw);
    roll = atan2(V.*yawrate,g);
end

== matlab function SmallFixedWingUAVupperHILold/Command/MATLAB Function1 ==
function xdx  = track(x,t,sample_tt)
%     index = int8(t/sample_tt);
%     if index <= 1
%         index = int8(1);
%     end
%     if index >= length(x)
%         index = int8(length(x));
%     end
    index = 1;
    xx = x(index+100);
    yy = x(index+200);

    xdx = [xx;-yy;0];
end

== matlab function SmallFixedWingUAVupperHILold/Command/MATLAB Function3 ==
function [av1,Hz,yaw,roll] = DF(xd,dxd,ddxd,x,dx,g)
    av1 = (0); 
    Hz= (0); 
    yaw= (0); 
    roll= (0); 
    xd = [xd(1);xd(2);xd(3)];
    dxd = [dxd(1);dxd(2);dxd(3)];
    ddxd = [ddxd(1);ddxd(2);ddxd(3)];
    x = [x(1);x(2);x(3)];
    dx = [dx(1);dx(2);dx(3)];
%     x1 = (xd-x)/norm(xd-x);
    r1 = zeros(3,1);
    r1 = (dxd+0.2*(xd-x))/(norm(dxd+0.2*(xd-x))+0.001);
    


    av1 = ( r1'*(1*ddxd-[0;0;g]+5*(dxd-dx)+3*(xd-x)));
     %%
%     t1 = zeros(3,1,'single');
%     t2 = zeros(3,1,'single');
%     t3 = zeros(3,1,'single');
%     t4 = zeros(3,1,'single');
%     t1(1,1) = ddxd(1,1);
%     t1(2,1) = ddxd(2,1);
%     t1(3,1) = ddxd(3,1) - single(g);
%     
%     for i = 1:3
%     t2(i,1) = single(3) * (dxd(i,1) - dx(i,1));
%     t3(i,1) = single(0.1) * (xd(i,1) - x(i,1));
% 
%     end
% 
%     for i = 1:3
%     t4(i,1) = t1(i,1) + t2(i,1) + t3(i,1);
%     end
%     av1 = single( r1'*t4);
%%

    an = (eye(3)-(r1*r1'))*((ddxd)-([0;0;g]));

    av3 = -(norm(an));
    
    Hz = (xd(3));


    r3 = (an)/((av3)+(0.001));

    r2 = cross(r3,r1);

    yaw = (atan2(r1(2),r1(1)));
    
    roll = (atan2(r2(3),r3(3)));

    if isnan(av1)
        av1=(0);
    end
    if isnan(Hz)
        Hz=(0);
    end
    if isnan(yaw)
        yaw=(0);
    end

end

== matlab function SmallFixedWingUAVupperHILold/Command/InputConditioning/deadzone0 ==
function y = fcn(u)
%Function description:
%  Control the range of the remote control input from RCMin to RCMax,which can be obtained from QGC. And set
%  a dead zone with a dead zone size of deadZone,the output y is normalized to 0~1.
RCMin = 1100;
RCMax = 1900;
RCMid = (RCMin + RCMax)/2;
deadZoneRate = 0.05;
deadZone = deadZoneRate*(RCMax - RCMin);
k = 1/(RCMax - RCMid - deadZone);
%Limiting
if(u < RCMin)
    u = RCMin;
elseif(u > RCMax)
    u = RCMax;
end
%dead zone and normalize
 if(u > RCMid + deadZone)
    y = (u-RCMid - deadZone)*k;
 elseif(u < RCMid - deadZone)
     y = (u - RCMid + deadZone)*k;
 else
     y = 0;
 end

 end

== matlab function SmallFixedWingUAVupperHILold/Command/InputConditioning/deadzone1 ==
function y = fcn(u)
%Function description:
%  Control the range of the remote control input from RCMin to RCMax, and set
%  a dead zone with a dead zone size of ±deadZone,the output y is
%  normalized to 0~1.You can get the RC calibration parameters in QGC.
RCMin = 1100;
RCMax = 1900;
RCMid = (RCMin + RCMax)/2;
deadZoneRate = 0.05;
deadZone = deadZoneRate*(RCMax - RCMin);
k = 1/(RCMax - RCMid - deadZone);
%Limiting
if(u < RCMin)
    u = RCMin;
elseif(u > RCMax)
    u = RCMax;
end
%dead zone and normalize
 if(u > RCMid + deadZone)
    y = (u-RCMid - deadZone)*k;
 elseif(u < RCMid - deadZone)
     y = (u - RCMid + deadZone)*k;
 else
     y = 0;
 end

 end

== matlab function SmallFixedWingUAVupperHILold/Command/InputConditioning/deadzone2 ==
function y = fcn(u)
%Function description:
%  Control the range of the remote control input from RCMin to RCMax, and set
%  a dead zone with a dead zone size of ±deadZone,the output y is
%  normalized to 0~1.You can get the RC calibration parameters in QGC.
RCMin = 1100;
RCMax = 1900;
RCMid = (RCMin + RCMax)/2;
deadZoneRate = 0.05;
deadZone = deadZoneRate*(RCMax - RCMin);
k = 1/(RCMax - RCMid - deadZone);
%Limiting
if(u < RCMin)
    u = RCMin;
elseif(u > RCMax)
    u = RCMax;
end
%dead zone and normalize
 if(u > RCMid + deadZone)
    y = (u-RCMid - deadZone)*k;
 elseif(u < RCMid - deadZone)
     y = (u - RCMid + deadZone)*k;
 else
     y = 0;
 end

 end
